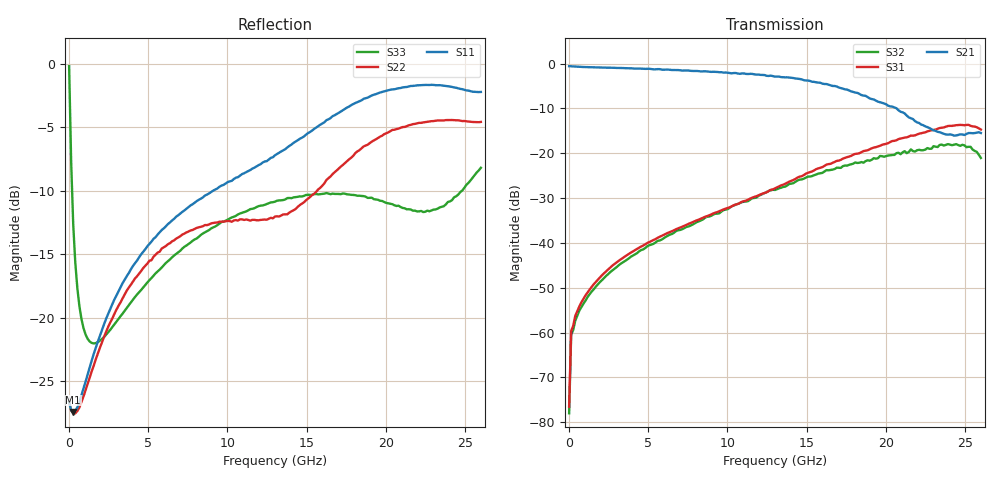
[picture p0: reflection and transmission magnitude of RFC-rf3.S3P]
!  3-Port S-parameters saved by WinCal
! VAR MeasName=S-Parameters (CALIBRATED_DATA) read from VNA (N5245A)
! VAR MeasDate=2016-7-4 10:45:17
! VAR NAME=25_C168105_RF2_RF3_01
! VAR FILENAME=25_C168105_RF2_RF3_01.S3P
! VAR DATE=2016-7-4 10:45:17
! VAR PHYS_PORTS=1,2,3
# Hz S DB R 50
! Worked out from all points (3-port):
!   201 points, 10 MHz to 26 GHz, reference 50 ohm
!   strongest paths, dB at 10 MHz, 6.508 GHz, 13.01 GHz, 19.5 GHz, 26 GHz:
!     S21: -0.6, -1.4, -2.9, -8.5, -15.5
!     S31: -76.5, -37.4, -27.8, -18.5, -14.7
!     S32: -78.0, -38.0, -28.2, -21.1, -21.0
!   lowest |S11| = -27.4 dB at 269.9 MHz (marker M1), VSWR 1.09, Z = 53.7 - j2.33 ohm
!   |S11| at or under -10 dB: start of sweep to 9.099 GHz
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1e7  -26.67 -3.4  -0.58 -0.3  -80.93 60.6
     -0.58 -0.3  -26.64 -5.0  -73.03 60.0
     -76.55 42.2  -78.01 51.3  -0.18 -9.3
1.3995e8  -27.32 -17.6  -0.62 -2.0  -59.30 46.3
          -0.61 -2.1  -27.35 -15.6  -60.39 45.1
          -59.66 46.7  -60.50 48.4  -7.78 -66.2
2.699e8  -27.44 -30.6  -0.65 -3.7  -58.77 39.6
         -0.64 -3.8  -27.51 -27.1  -59.83 37.1
         -58.44 41.9  -59.38 40.1  -12.69 -78.2
6.5975e8  -26.67 -58.4  -0.73 -8.4  -54.13 51.8
          -0.72 -8.5  -27.09 -52.4  -55.09 49.8
          -54.14 51.2  -55.05 49.8  -19.11 -88.5
1.43945e9  -23.37 -87.2  -0.83 -17.4  -49.78 58.7
           -0.82 -17.5  -24.22 -79.7  -50.86 55.0
           -49.78 58.7  -50.84 55.3  -22.00 -96.1
6.7674e9  -12.05 -166.2  -1.45 -79.0  -36.97 49.6
          -1.41 -78.7  -13.77 -154.4  -37.39 32.4
          -36.93 49.9  -37.32 32.8  -14.98 -134.0
1.3005e10  -7.20 138.8  -2.98 -152.6  -27.96 18.9
           -2.91 -153.1  -12.04 94.5  -28.42 -27.8
           -27.83 18.1  -28.20 -27.8  -10.86 174.7
1.807305e10  -3.09 96.4  -6.92 137.8  -20.60 -34.4
             -6.46 140.3  -7.03 -33.8  -22.14 -93.7
             -20.14 -33.2  -22.06 -94.4  -10.35 122.9
2.145175e10  -1.78 62.7  -11.86 111.1  -16.36 -76.4
             -12.01 105.8  -4.84 -90.7  -19.76 -151.8
             -16.28 -79.3  -19.71 -149.4  -11.46 84.6
2.6e10  -2.21 27.9  -15.32 104.1  -14.81 -172.8
        -15.49 100.6  -4.58 -136.6  -21.31 110.6
        -14.71 -175.7  -21.05 112.0  -8.19 34.1
